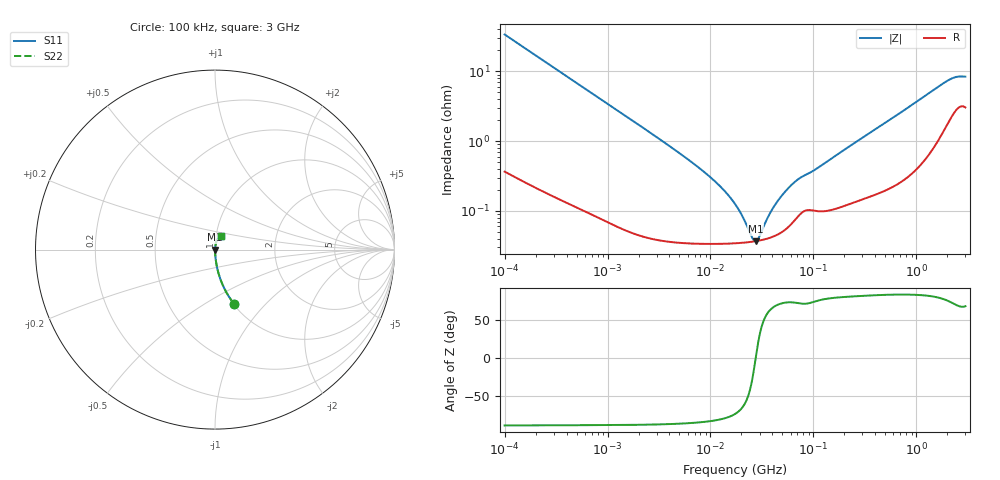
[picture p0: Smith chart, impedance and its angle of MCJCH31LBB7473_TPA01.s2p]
! MCJCH31LBB7473_TPA01  S-PARAMETER MODEL  ( Standard Model )
! Model Generated by TAIYO YUDEN Corporation (http://www.ty-top.com)
! Version 1.0
! TAIYO YUDEN Control No. 220601
! Copyright(c) 2015 TAIYO YUDEN CO.,LTD. All Rights Reserved.
! Product Description (link to TY-COMPAS)
! https://ds.yuden.co.jp/TYCOMPAS/or/detail?pn=MCJCH31LBB7473KTPA01&u=M
! Products Name : Multilayer Ceramic Capacitors
! Characteristics :
!  Capacitance : 0.047 [uF] , Rated Voltage : 100 [V] , TCC : X7R
!  Case Size : 3.2 x 1.6 / 0.126 x 0.063 [mm/inch] , Thickness : 1.6 / 0.063 [mm/inch]
!  (Conditions: Temperature = 25 [degC] , DC Bias Voltage = 0 [V])
! External Node Assignments :
!  1  o---| |---o  2
! GND o---------o GND
! Frequency Range : 100kHz  -  3GHz  [ 401 STEP ]
# MHZ S RI R 50
! Freq[MHz].  S11 Real  S11 Imag  S21 Real  S21 Imag  S12 Real  S12 Imag  S22 Real  S22 Imag
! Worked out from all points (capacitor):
!   401 points, 100 kHz to 3 GHz, reference 50 ohm
!   read as one part in series: C = 46.9 nF near 105.3 kHz
!   lowest |Z| = 36.8 mohm at 27.54 MHz (marker M1)
!   series resonance near 27.51 MHz, so ESL is about 710 pH
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0.1  0.1056 -0.302  0.8944 0.302  0.8944 0.302  0.1056 -0.302
0.147195  0.0529 -0.218  0.9471 0.218  0.9471 0.218  0.0529 -0.218
0.228123  0.0236 -0.1456  0.9764 0.1456  0.9764 0.1456  0.0236 -0.1456
0.562235  0.00473 -0.0607  0.9953 0.0607  0.9953 0.0607  0.00473 -0.0607
3.161081  0.000496 -0.0108  0.9995 0.0108  0.9995 0.0108  0.000496 -0.0108
6.178009  0.00037 -0.00534  0.9996 0.00534  0.9996 0.00534  0.00037 -0.00534
9.824692  0.000346 -0.00309  0.9997 0.00309  0.9997 0.00309  0.000346 -0.00309
13.7349  0.000342 -0.0019  0.9997 0.0019  0.9997 0.0019  0.000342 -0.0019
17.7727  0.000345 -0.00114  0.9997 0.00114  0.9997 0.00114  0.000345 -0.00114
20.74485  0.00035 -0.000724  0.9996 0.000724  0.9996 0.000724  0.00035 -0.000724
25.49486  0.000362 -0.000193  0.9996 0.000193  0.9996 0.000193  0.000362 -0.000193
27.54426  0.000368 2.85e-06  0.9996 -2.85e-06  0.9996 -2.85e-06  0.000368 2.85e-06
29.75839  0.000376 0.000199  0.9996 -0.000199  0.9996 -0.000199  0.000376 0.000199
35.64176  0.000401 0.000666  0.9996 -0.000666  0.9996 -0.000666  0.000401 0.000666
39.51212  0.000422 0.000943  0.9996 -0.000943  0.9996 -0.000943  0.000422 0.000943
49.82709  0.000503 0.00161  0.9995 -0.00161  0.9995 -0.00161  0.000503 0.00161
67.88584  0.000779 0.00258  0.9992 -0.00258  0.9992 -0.00258  0.000779 0.00258
97.38194  0.00103 0.00353  0.999 -0.00353  0.999 -0.00353  0.00103 0.00353
547.5153  0.00247 0.0198  0.9975 -0.0198  0.9975 -0.0198  0.00247 0.0198
1986.261  0.0215 0.0682  0.9785 -0.0682  0.9785 -0.0682  0.0215 0.0682
2441.062  0.0328 0.0739  0.9672 -0.0739  0.9672 -0.0739  0.0328 0.0739
3000  0.0352 0.0735  0.9648 -0.0735  0.9648 -0.0735  0.0352 0.0735
